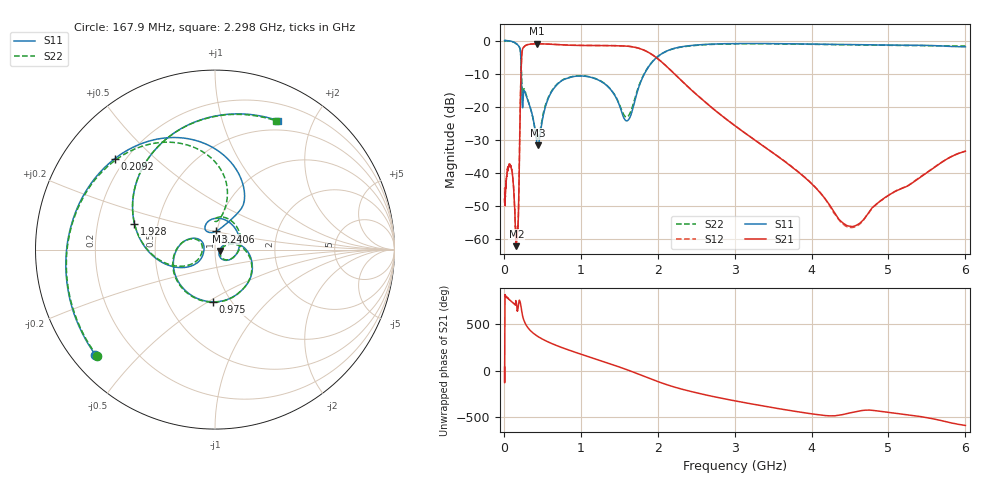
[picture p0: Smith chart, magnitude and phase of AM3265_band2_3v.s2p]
!Agilent Technologies,E8364B,MY43040894,A.07.50.67
!Agilent E8364B: A.07.50.67
!Date: Friday, May 09, 2025 07:23:41
!Correction: S11(Full 2 Port(1,2))
!S21(Full 2 Port(1,2))
!S12(Full 2 Port(1,2))
!S22(Full 2 Port(1,2))
!S2P File: Measurements: S11, S21, S12, S22:Log Frequency Sweep
# Hz S  dB  R 50
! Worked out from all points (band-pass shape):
!   3201 points, 10 MHz to 6 GHz, reference 50 ohm
!   highest |S21| = -0.99 dB at 430.4 MHz (marker M1); lowest = -62.1 dB at 162.9 MHz (marker M2)
!   |S21| within 3 dB of the highest: 234.8 MHz to 1.909 GHz (1.674 GHz wide, 156 % of centre)
!   lowest |S11| = -31.6 dB at 443.5 MHz (marker M3), VSWR 1.05, Z = 52.6 - j0.724 ohm
!   |S11| at or under -10 dB: 226.6 MHz to 1.829 GHz (1.602 GHz wide, 156 % of centre)
!   |S22| runs from -29.8 to 0.0 dB; largest |S21 - S12| = 0.0098
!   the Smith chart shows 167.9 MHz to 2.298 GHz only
!   S11 on the Smith chart (normalised r, x): 167.9 MHz: 0.07, -0.38; 209.2 MHz: 0.16, +0.38; 240.6 MHz: 0.99, +0.20; 975 MHz: 0.83, -0.53; 1.928 GHz: 0.37, +0.14; 2.298 GHz: 0.38, +1.54
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1e7  -0.03 -6.5  -47.90 38.6  -44.71 -152.6  -0.07 -6.3
2.908064e7  -0.04 -18.6  -42.64 73.6  -42.49 73.3  -0.04 -18.7
8.439949e7  -0.16 -56.6  -37.82 32.4  -37.78 33.2  -0.20 -56.8
1.629178e8  -0.94 -132.0  -62.11 7.3  -59.17 -135.2  -0.98 -131.5
1.678769e8  -1.04 -138.6  -60.30 -20.3  -59.38 -166.6  -1.06 -138.1
2.091655e8  -2.45 137.9  -24.71 24.1  -24.70 24.2  -2.40 143.0
2.405814e8  -19.90 88.0  -2.88 -119.3  -2.85 -119.3  -15.55 82.8
2.44949e8  -20.27 102.2  -2.50 -136.2  -2.46 -136.2  -16.12 88.3
3.126026e8  -18.11 -8.5  -1.23 101.1  -1.19 101.0  -18.04 -9.1
4.304277e8  -30.91 -35.5  -0.99 13.1  -0.96 13.1  -29.48 -27.7
4.435298e8  -31.60 -15.2  -0.99 6.1  -0.96 6.1  -29.71 -11.8
7.123273e8  -12.87 -23.6  -1.28 -99.2  -1.24 -99.2  -12.74 -27.2
9.749507e8  -10.72 -92.0  -1.49 -175.9  -1.46 -176.0  -10.63 -94.5
1.3505e9  -13.86 175.1  -1.54 81.9  -1.51 81.8  -13.79 175.0
1.927655e9  -6.53 162.1  -4.27 -94.1  -4.24 -94.1  -6.47 161.4
2.067357e9  -3.79 121.5  -6.80 -136.3  -6.78 -136.2  -3.79 121.7
2.298416e9  -1.94 63.9  -11.92 165.1  -11.89 165.1  -2.01 64.8
3.202913e9  -0.90 -91.5  -29.08 6.0  -29.07 5.9  -0.97 -91.5
3.818953e9  -1.01 -178.2  -39.52 -80.3  -39.46 -80.4  -1.09 -179.7
4.490206e9  -1.21 91.9  -56.06 -94.6  -56.45 -99.9  -1.30 90.5
5.185309e9  -1.41 1.1  -44.55 -107.9  -44.49 -108.5  -1.52 1.3
6e9  -1.92 -96.9  -33.43 132.5  -33.43 132.5  -1.69 -96.5
